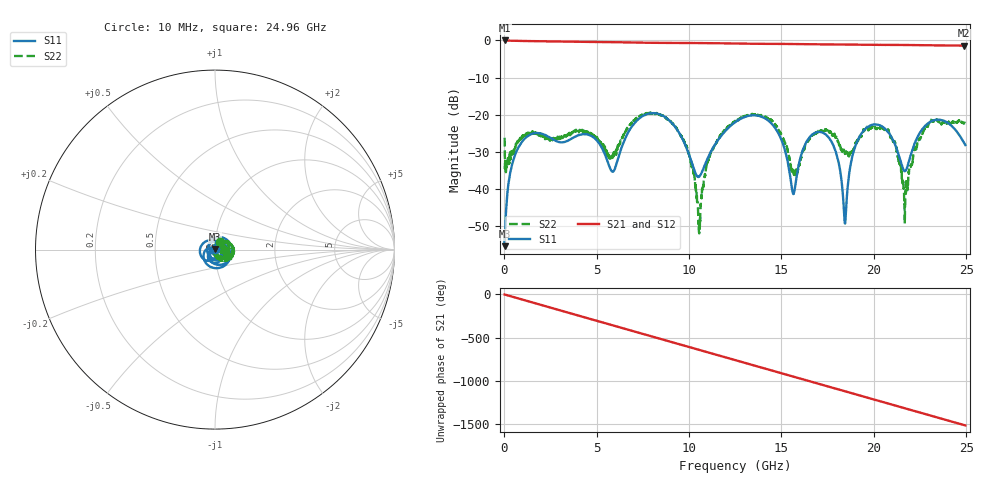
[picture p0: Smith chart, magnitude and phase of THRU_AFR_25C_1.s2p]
!Keysight Technologies,M9372A,MY54321388,A.12.55.09
!Automatic Fixture Removal (AFR)
!Date: Wednesday, May 22, 2019 8:33:19 AM
!S2P File: Measurements: S11,S21,S12,S22:
# MHz S  RI  R 50
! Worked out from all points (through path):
!   2496 points, 10 MHz to 24.96 GHz, reference 50 ohm
!   highest |S21| = -0.01 dB at 40 MHz (marker M1); lowest = -1.4 dB at 24.89 GHz (marker M2)
!   group delay of S21, straight-line fit = 168 ps
!   lowest |S11| = -55.4 dB at 20 MHz (marker M3), VSWR 1.00, Z = 50 + j0.167 ohm
!   |S11| at or under -10 dB: start of sweep to end of sweep
!   |S22| runs from -51.9 to -19.4 dB; largest |S21 - S12| = 1.4e-15
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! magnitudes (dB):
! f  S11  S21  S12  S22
! 10 MHz  -52.6  -0.1  -0.1  -26.2
! 20 MHz  -55.4  0.0  0.0  -29.0
! 40 MHz  -51.3  0.0  0.0  -32.4
! 1.03 GHz  -26.8  -0.2  -0.2  -25.5
! 4.17 GHz  -25.3  -0.4  -0.4  -24.0
! 5.87 GHz  -35.3  -0.5  -0.5  -31.5
! 8.33 GHz  -19.8  -0.7  -0.7  -19.7
! 9.82 GHz  -28.4  -0.7  -0.7  -28.2
! 10.55 GHz  -36.7  -0.7  -0.7  -51.9
! 11.1 GHz  -30.7  -0.7  -0.7  -31.8
! 12.49 GHz  -22.0  -0.8  -0.8  -21.6
! 14.51 GHz  -22.6  -0.9  -0.9  -21.7
! 15.65 GHz  -41.3  -1.0  -1.0  -34.9
! 16.65 GHz  -25.4  -1.0  -1.0  -25.5
! 17.81 GHz  -28.2  -1.1  -1.1  -25.5
! 18.44 GHz  -49.2  -1.1  -1.1  -30.6
! 19.25 GHz  -25.7  -1.1  -1.1  -25.7
! 20.81 GHz  -24.9  -1.2  -1.2  -24.7
! 21.73 GHz  -35.0  -1.2  -1.2  -40.3
! 23.01 GHz  -22.1  -1.3  -1.3  -22.1
! 24.89 GHz  -27.6  -1.4  -1.4  -22.1
! 24.96 GHz  -28.1  -1.4  -1.4  -22.2
